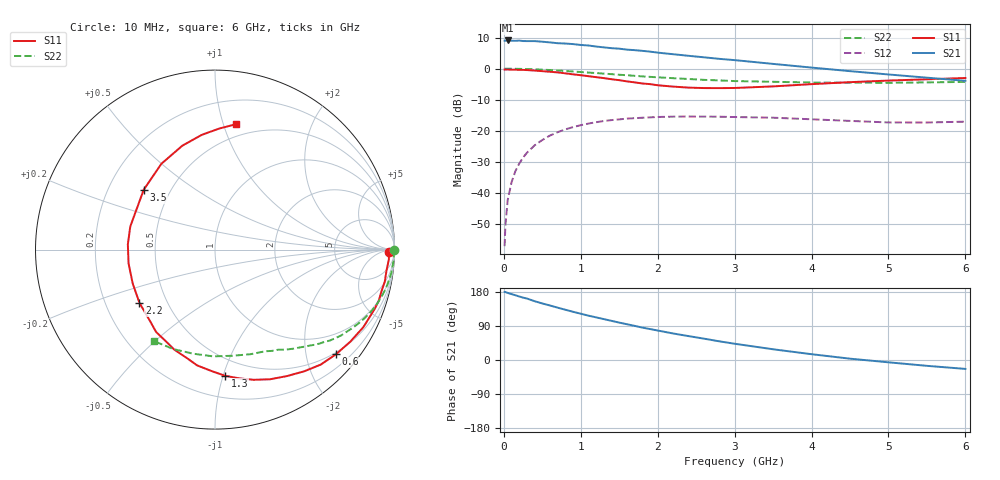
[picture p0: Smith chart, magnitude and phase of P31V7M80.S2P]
! SIEMENS Small Signal Semiconductors
! BFP181
! Si NPN RF Bipolar Junction Transistor in SOT143
! VCE = 1.75 V  IC = 0.8 mA
! Common Emitter S-Parameters:  March  1996
# GHz  S  MA  R  50
!  f  S11  S21  S12  S22
! GHz  MAG  ANG  MAG  ANG  MAG  ANG  MAG  ANG
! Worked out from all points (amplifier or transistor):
!   36 points, 10 MHz to 6 GHz, reference 50 ohm
!   highest |S21| = 9.1 dB at 50 MHz (marker M1)
!   |S21| within 3 dB of that: start of sweep to 1.629 GHz
!   unconditionally stable (mu >= 1): 3.312 GHz to end of sweep
!   at 250 MHz: K = 0.09, MSG = 18.7 dB, |S12| = -28.6 dB
!   at 1.4 GHz: K = 0.47, MSG = 11.6 dB, |S12| = -16.5 dB
!   at 6 GHz: K = 1.36, MAG = 3.0 dB, |S12| = -17.0 dB
!   S11 on the Smith chart (normalised r, x): 10 MHz: 50, -24; 600 MHz: 0.46, -2.62; 1.3 GHz: 0.36, -1.01; 2.2 GHz: 0.35, -0.28; 3.5 GHz: 0.35, +0.32; 6 GHz: 0.39, +1.10
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0.01  0.9681 -0.9  2.814 179.7  0.0014 87.7  0.9994 -0.2
0.02  0.9685 -1.6  2.806 179.4  0.003 89.1  0.9983 -0.7
0.05  0.9704 -3.2  2.841 177.0  0.0077 88.6  0.9968 -1.6
0.1  0.9625 -7.0  2.811 173.9  0.0149 84.0  0.9974 -3.3
0.15  0.9627 -10.7  2.803 170.9  0.0225 82.4  0.9944 -4.9
0.2  0.9564 -13.8  2.826 167.6  0.0298 80.9  0.9926 -6.5
0.25  0.9557 -17.4  2.78 164.6  0.0372 78.2  0.9892 -8.2
0.4  0.9327 -27.6  2.774 155.2  0.0585 71.4  0.9765 -12.9
0.6  0.8915 -40.8  2.642 143.8  0.0841 62.5  0.9504 -19.0
0.9  0.8106 -60.4  2.483 127.2  0.115 50.3  0.8999 -27.1
1.1  0.757 -73.4  2.357 117.0  0.1311 43.0  0.8652 -31.9
1.3  0.705 -85.5  2.201 107.9  0.1441 36.4  0.8327 -36.3
1.5  0.6527 -98.8  2.097 98.7  0.1528 30.8  0.7976 -40.1
1.8  0.5778 -118.8  1.934 85.5  0.1626 23.2  0.7518 -45.3
2.2  0.515 -144.8  1.707 70.0  0.1692 14.4  0.7034 -51.7
2.8  0.4864 176.6  1.438 49.3  0.1689 4.3  0.6477 -60.6
3  0.4892 164.8  1.372 42.9  0.1668 1.3  0.6318 -63.7
3.5  0.5186 140.0  1.193 28.3  0.1628 -3.7  0.615 -71.5
4  0.5638 122.0  1.041 15.3  0.1535 -7.5  0.5992 -80.8
4.5  0.6067 107.5  0.912 3.5  0.1446 -9.4  0.5949 -91.1
5.5  0.6744 88.1  0.716 -15.4  0.1362 -5.7  0.601 -112.7
6  0.7079 80.6  0.638 -23.5  0.1406 -3.6  0.6127 -123.8
